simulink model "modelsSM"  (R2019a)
settings: Solver=VariableStepAuto  StartTime=0.0  StopTime=10.0  RelTol=1e-3
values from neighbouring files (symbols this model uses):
  c = 8e-3    (= 0.008)    [initParams.m]
  g = 9.81    [initParams.m]
  L1 = 0.5    [initParams.m]
  m = 0.2    [initParams.m]
  R = 10    [initParams.m]
  x0 = [0.1;0;0.3]    [initParams.m]

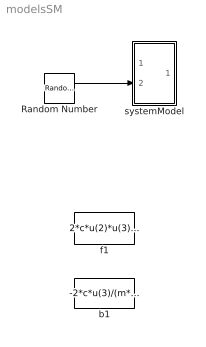
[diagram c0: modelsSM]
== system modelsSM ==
  Random Number : RandomNumber  Variance=1e-3  SampleTime=0.01
  b1 : Fcn  Expr=-2*c*u(3)/(m*L1*u(1)^2)
  f1 : Fcn  Expr=2*c*u(2)*u(3)^2/(m*u(1)^3)-2*c*u(3)*(2*c*u(2)*u(3)/(L1*u(1)^2)-R*u(3)/L1)/(m*u(1)^2)
  systemModel : Subsystem
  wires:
  Random Number/1 -> systemModel/2("d ")

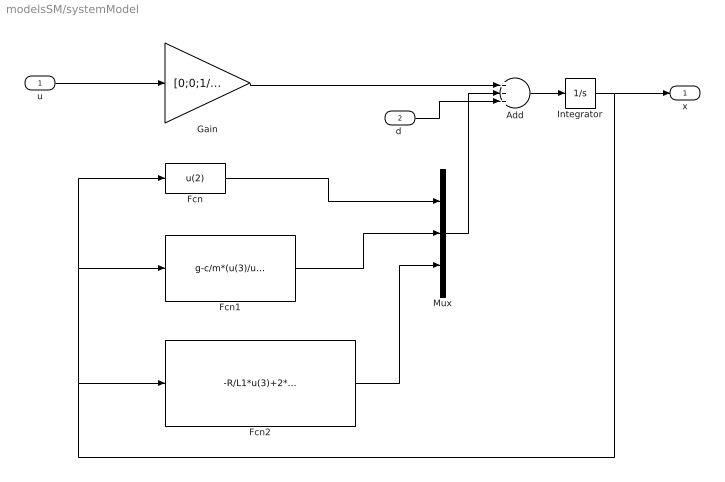
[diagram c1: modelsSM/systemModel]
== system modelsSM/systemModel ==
  u : Inport
  "d " : Inport  Port=2
  Add : Sum  Inputs=+++
  Fcn : Fcn  Expr=u(2)
  Fcn1 : Fcn  Expr=g-c/m*(u(3)/u(1))^2
  Fcn2 : Fcn  Expr=-R/L1*u(3)+2*c/L1*(u(2)*u(3)/(u(1))^2)
  Gain : Gain  Gain=[0;0;1/L1]  Multiplication=Matrix(K*u) (u vector)
  Integrator : Integrator  InitialCondition=x0
  Mux : Mux  Inputs=3
  x : Outport
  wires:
  Integrator/1 -> x/1, Fcn/1, Fcn1/1, Fcn2/1
  Gain/1 -> Add/1
  Fcn/1 -> Mux/1
  Fcn1/1 -> Mux/2
  Mux/1 -> Add/2
  Fcn2/1 -> Mux/3
  u/1 -> Gain/1
  Add/1 -> Integrator/1
  "d "/1 -> Add/3
